FUNCTION_BLOCK FB_SeparatingModule EXTENDS FB_Module
// Module to separate via sensor, barrier and clamp cylinder and axis
VAR_INPUT
		(***** Information about the state and mode of machine *****)
	bExecute					: BOOL;
	bSemiStart					: BOOL;
		(****** Variables to enable / disable diagnosis and temperature mode ******)
	bClampDiag					: BOOL;
	bClampTemp					: BOOL;
	bClampRecord				: BOOL;
	bBarrierDiag				: BOOL;
	bBarrierTemp				: BOOL;
	bBarrierRecord				: BOOL;
		(***** Timer values for clamp and barrier cylinder *****)
	tTimeOutClamp				: TIME;
	tTimeOutBarrier				: TIME;
	tRecordIntervallClamp		: TIME;
	tRecordIntervallBarrier		: TIME;
	tBarrierAtWork				: TIME;
		(***** Information about number of boxes being sorted *****)
	iBoxesOnTheWay				: INT;
		(***** Buttons *****)
	bButtonClampToWorkIn		: BOOL;
	bButtonClampToBaseIn		: BOOL;
	bButtonBarrierToWorkIn		: BOOL;
	bButtonBarrierToBaseIn		: BOOL;
END_VAR
VAR_OUTPUT
	bClampToWork				: BOOL;
	bClampAtBase				: BOOL;
	bClampAtWork				: BOOL;
	bBarrierToWork				: BOOL;
	bBarrierAtBase				: BOOL;
	bBarrierAtWork				: BOOL;
	bClampError					: BOOL;
	sClampErrorMsg				: STRING;
	bBarrierError				: BOOL;
	sBarrierErrorMsg			: STRING;
	aClampTemps					: ARRAY[1..100] OF LREAL;
	aBarrierTemps				: ARRAY[1..100] OF LREAL;
	bSeparated					: BOOL;
	bButtonClampToWorkOut		: BOOL;
	bButtonClampToBaseOut		: BOOL;
	bButtonBarrierToWorkOut		: BOOL;
	bButtonBarrierToBaseOut		: BOOL;
END_VAR
VAR
(* ================= Function block and interface instances ===================== *)
	
	fbSensor					: FB_SignalHandling;
	
		(* Instances of clamp cylinder function blocks *)
	fbClamp						: FB_Cylinder;					// Without diagnosis and temperature mode
	fbClampDiag					: FB_CylinderDiag;				// With diagnosis of states
	fbClampTemp					: FB_CylinderTemp;				// With temperature mode
	fbClampTempDiag				: FB_CylinderTempDiag;			// With diagnosis of temperature
	fbClampTempRecord			: FB_CylinderTempRecord;		// With record of temperatures
		(* Interface instance of ICylinder for clamp cylinder *)
	iClamp						: ICylinder;
	
			(* Instances of barrier cylinder function blocks *)
	fbBarrier					: FB_Cylinder;					// Without diagnosis and temperature mode
	fbBarrierDiag				: FB_CylinderDiag;				// With diagnosis of states
	fbBarrierTemp				: FB_CylinderTemp;				// With temperature mode
	fbBarrierTempDiag			: FB_CylinderTempDiag;			// With diagnosis of temperature
	fbBarrierTempRecord			: FB_CylinderTempRecord;		// With record of temperatures
		(* Interface instance of ICylinder for barrier cylinder *)
	iBarrier					: ICylinder;
	
				(***** Manual cylinder control *****)
	fbButtonClampToWork			: FB_SignalHandlingIntern;		// To move manually clamp cylinder to work position
	fbButtonClampToBase			: FB_SignalHandlingIntern;		// To move manually clamp cylinder to base position
	fbButtonBarrierToWork		: FB_SignalHandlingIntern;		// To move manually barrier cylinder to work position
	fbButtonBarrierToBase		: FB_SignalHandlingIntern;		// To move manually barrier cylinder to base position
	
(* ========================== COMMON VARIABLES =============================== *)	
	fbTimerBarrierAtWork		: TON;							// Timer for opening barrier in AUTOMATIC mode
	eStateAuto					: E_StateSeparatingAuto;
	eStateSemiAuto				: E_StateSeparatingAuto;
END_VAR

// =========================================================
;
// =========================================================

METHOD PROTECTED M_ResetState
VAR_INPUT
END_VAR
// =========================================================

eStateAuto 		:= eSeparatingAuto_Init;
eStateSemiAuto	:= eSeparatingAuto_Init;

// =========================================================
END_METHOD

METHOD PUBLIC M_Semiautomatic
VAR_INPUT
END_VAR
// =========================================================
	// Noticing work position of barrier cylinder	

fbTimerBarrierAtWork( PT := tBarrierAtWork );

// =========================================================
	// Control of main axis

IF iBoxesOnTheWay = 0 AND eStateSemiAuto = eSeparatingAuto_Init THEN
	bHalt := TRUE;
	M_Stop();
END_IF

IF bHalt THEN
	IF bHaltDone THEN
		bHalt := FALSE;
	END_IF
	
	M_Stop();
ELSE
	fbAxis.M_MoveFw();
END_IF

// =========================================================
	// Process of separating boxes
	
CASE eStateSemiAuto OF
	// =========================================================
	eSeparatingAuto_Init:
	
			iBarrier.M_MoveToBase();					(***** Calling method of FB via interface *****)
			
			IF iBarrier.P_AtBasePos						(***** Accessing property of FB via interface *****)
			AND bExecute AND bSemiStart THEN
				eStateSemiAuto := eSeparatingAuto_Start;
			END_IF
		
	// =========================================================
	eSeparatingAuto_Start:
	
			IF fbSensor.bOut THEN
				eStateSemiAuto := eSeparatingAuto_CloseClamp;
			ELSE
				IF NOT iClamp.P_AtWorkPos THEN			(***** Accessing property of FB via interface instance *****)
					iClamp.M_MoveToWork();				(***** Calling method of FB via interface instance *****)
				END_IF
				
				fbAxis.M_MoveFw();
			END_IF
		
	// =========================================================
	eSeparatingAuto_CloseClamp:
	
			iClamp.M_MoveToBase();						(***** Calling method of FB via interface instance *****)
			
			IF iClamp.P_AtBasePos THEN					(***** Accessing property of FB via interface instance *****)
				bSeparated 		:= TRUE;
				eStateSemiAuto 	:= eSeparatingAuto_OpenBarrier;
			END_IF
		
	// =========================================================
	eSeparatingAuto_OpenBarrier:
	
			iBarrier.M_MoveToWork();					(***** Calling method of FB via interface *****)
			
			IF iBarrier.P_AtWorkPos THEN				(***** Accessing property of FB via interface *****)
				fbTimerBarrierAtWork( IN := TRUE );
			END_IF
			
			IF fbTimerBarrierAtWork.Q THEN
				fbTimerBarrierAtWork( IN := FALSE );
				eStateSemiAuto := eSeparatingAuto_CloseBarrier;
			END_IF
		
	// =========================================================
	eSeparatingAuto_CloseBarrier:
	
			iBarrier.M_MoveToBase();					(***** Calling method of FB via interface *****)
			
			IF iBarrier.P_AtBasePos THEN				(***** Accessing property of FB via interface *****)
				bSeparated 		:= FALSE;
				eStateSemiAuto 	:= eSeparatingAuto_OpenClamp;
			END_IF
		
	// =========================================================
	eSeparatingAuto_OpenClamp:
	
			iClamp.M_MoveToWork();						(***** Calling method of FB via interface instance *****)
			
			IF iClamp.P_AtWorkPos THEN					(***** Accessing property of FB via interface instance *****)
				eStateSemiAuto := eSeparatingAuto_Init;
			END_IF
END_CASE

// =========================================================
END_METHOD

METHOD PUBLIC M_SetOutput
VAR_INPUT
END_VAR
// =========================================================
		// Calling method M_SetOutput of base class FB_Module via 'SUPER^.'
		
SUPER^.M_SetOutput();						

// =========================================================
		// Sensor
		
fbSensor.M_SetOutput();

// =========================================================
		// Cylinder buttons
		
fbButtonClampToWork.M_SetOutput();
fbButtonClampToBase.M_SetOutput();
fbButtonBarrierToWork.M_SetOutput();
fbButtonBarrierToBase.M_SetOutput();

// =========================================================
		// Output variables for cylinders
		
bClampToWork 	:= iClamp.P_ToWork;			// Assigning global output variable to property of selected FB
											// Accessing property of selected FB via interface instance
bClampAtWork 	:= iClamp.P_AtWorkPos;
bClampAtBase 	:= iClamp.P_AtBasePos;
		
bBarrierToWork 	:= iBarrier.P_ToWork;		// Assigning global output variable to property of selected FB
											// Accessing property of selected FB via interface instance
bBarrierAtWork 	:= iBarrier.P_AtWorkPos;
bBarrierAtBase	:= iBarrier.P_AtBasePos;

// =========================================================
		// Buttons

fbButtonClampToWork.bInput 		:= bButtonClampToWorkIn;
fbButtonClampToBase.bInput 		:= bButtonClampToBaseIn;
fbButtonBarrierToWork.bInput 	:= bButtonBarrierToWorkIn;
fbButtonBarrierToBase.bInput 	:= bButtonBarrierToBaseIn;
bButtonClampToWorkOut 			:= fbButtonClampToWork.bOut;
bButtonClampToBaseOut 			:= fbButtonClampToBase.bOut;
bButtonBarrierToWorkOut 		:= fbButtonBarrierToWork.bOut;
bButtonBarrierToBaseOut 		:= fbButtonBarrierToBase.bOut;

// =========================================================
END_METHOD

METHOD PUBLIC M_Manual
VAR_INPUT
END_VAR
// =========================================================
	// Calling method M_Manual of base class FB_Module via 'SUPER^.'
		
SUPER^.M_Manual();							

// =========================================================
	// Manual cylinder control
	
IF fbButtonClampToWork.bOut THEN
	iClamp.M_MoveToWork();					(**** Calling method of FB via interface instance ****)
	
ELSIF fbButtonClampToBase.bOut THEN
	iClamp.M_MoveToBase();					(**** Calling method of FB via interface instance ****)
END_IF

IF fbButtonBarrierToWork.bOut THEN
	iBarrier.M_MoveToWork();				(**** Calling method of FB via interface instance ****)
	
ELSIF fbButtonBarrierToBase.bOut THEN
	iBarrier.M_MoveToBase();				(**** Calling method of FB via interface instance ****)
END_IF

// =========================================================
END_METHOD

METHOD PUBLIC M_Reset
VAR_INPUT
END_VAR
// =========================================================
		// Resetting cylinder and axis
		
fbTriggerResetStart( CLK := bReset );

IF fbTriggerResetStart.Q THEN
	bSeparated := FALSE;
	
	fbTimerBarrierAtWork( IN := FALSE );
	iClamp.M_Reset();					(**** Calling method of FB via interface ****)
	iBarrier.M_Reset();					(**** Calling method of FB via interface ****)
END_IF

// =========================================================
		// Calling method of base class
		
SUPER^.M_Reset();						// Calling method M_Reset of base class FB_Module via 'SUPER^.'

// =========================================================
END_METHOD

METHOD PUBLIC M_Maintenance
VAR_INPUT
END_VAR
// =========================================================
	// Calling own method M_Manual of this class FB_SeparatingModule via 'THIS^.'
		
THIS^.M_Manual();				

// =========================================================
END_METHOD

METHOD PUBLIC M_Enable
VAR_INPUT
END_VAR
// =========================================================
		// Calling method M_Enable of base class FB_Module via 'SUPER^.'
		
SUPER^.M_Enable();

// =========================================================
		// Sensor control
		
fbSensor.bEnable := bSensorEnable;

// =========================================================
		// Cylinder control
		
fbButtonClampToWork.bEnable		:= bManualCylinderEnable
									AND NOT iClamp.P_AtWorkPos;		(*** Accessing property of FB via interface instance ***)
								
fbButtonClampToBase.bInput 		:= NOT fbButtonClampToWork.bInput;

fbButtonClampToBase.bEnable 	:= bManualCylinderEnable
									AND NOT iClamp.P_AtBasePos;		(*** Accessing property of FB via interface instance ***)

fbButtonBarrierToWork.bEnable 	:= bManualCylinderEnable
									AND NOT iBarrier.P_AtWorkPos;	(*** Accessing property of FB via interface instance ***)
								
fbButtonBarrierToBase.bInput 	:= NOT fbButtonBarrierToWork.bInput;

fbButtonBarrierToBase.bEnable 	:= bManualCylinderEnable
									AND NOT iBarrier.P_AtBasePos;	(*** Accessing property of FB via interface instance ***)

// =========================================================
END_METHOD

METHOD PUBLIC M_CylinderOptions
VAR_INPUT
END_VAR
// =========================================================
		// Selecting clamp cylinder

// Checking variables to enable / disable diagnosis and temperature mode
IF bClampDiag THEN
	IF bClampTemp THEN
		
	(* ============== FB with diagnosis and temperature mode ============== *)
		bClampError 	:= fbClampTempDiag.bError;			// Assigning global output variable to output variable of selected FB
		sClampErrorMsg 	:= fbClampTempDiag.sErrorMsg;
		iClamp 			:= fbClampTempDiag;					// Assigning desired FB instance to interface instance
	
	ELSE
	
	(* ============== FB with diagnosis and without temperature mode ============== *)
		fbClampDiag.tTimeOut 	:= tTimeOutClamp;			// Setting special data for selected FB
		bClampError 			:= fbClampDiag.bError;		// Assigning global output variable to output variable of selected FB
		sClampErrorMsg 			:= fbClampDiag.sErrorMsg;
		iClamp 					:= fbClampDiag;				// Assigning desired FB instance to interface instance
	END_IF
ELSE
	bClampError := FALSE;
	sClampErrorMsg := '';
	
	IF bClampTemp THEN
		IF bClampRecord THEN
			fbClampTempRecord.tIntervalTime 	:= tRecordIntervallClamp;	// Time of record interval
			fbClampTempRecord.bRecordStart 		:= bComprAirEnabled;		// Recording if compressed air is set
			
			fbClampTempRecord.M_Record();									// Calling method of function block FB_CylinderTempRecord
			
			aClampTemps 	:= fbClampTempRecord.aTemps;					// Saving output variable
			iClamp 			:= fbClampTempRecord;
		ELSE
			(* ============== FB without diagnosis and with temperature mode ============== *)
			iClamp := fbClampTemp; 						// Assigning desired FB instance to interface instance
		END_IF
	ELSE
	
	(* ============== FB without diagnosis and temperature mode ============== *)
		iClamp := fbClamp;							// Assigning desired FB instance to interface instance						
	END_IF	
END_IF
									
// =========================================================
// =========================================================
			(**** Selecting barrier cylinder ****)

// Checking variables to enable / disable diagnosis and temperature mode
IF bBarrierDiag THEN
	IF bBarrierTemp THEN
		
	(* ============== FB with diagnosis and temperature mode ============== *)
		bBarrierError 		:= fbBarrierTempDiag.bError;		// Assigning global output variable to output variable of selected FB
		sBarrierErrorMsg 	:= fbBarrierTempDiag.sErrorMsg;
		iBarrier 			:= fbBarrierTempDiag;				// Assigning desired FB instance to interface instance
	
	ELSE
	
	(* ============== FB with diagnosis and without temperature mode ============== *)
		fbBarrierDiag.tTimeOut	:= tTimeOutBarrier;				// Setting special data for selected FB
		bBarrierError 			:= fbBarrierDiag.bError;		// Assigning global output variable to output variable of selected FB
		sBarrierErrorMsg 		:= fbBarrierDiag.sErrorMsg;
		iBarrier 				:= fbBarrierDiag;				// Assigning desired FB instance to interface instance
	END_IF
ELSE
	bBarrierError := FALSE;
	sBarrierErrorMsg := '';
	
	IF bBarrierTemp THEN
		IF bBarrierRecord THEN
			fbBarrierTempRecord.tIntervalTime 	:= tRecordIntervallBarrier;		// Time of record interval
			fbBarrierTempRecord.bRecordStart 	:= bComprAirEnabled;			// Recording if compressed air is set
			
			fbBarrierTempRecord.M_Record();										// Calling method of function block FB_CylinderTempRecord
			
			aBarrierTemps 	:= fbBarrierTempRecord.aTemps;						// Saving output variable
			iBarrier 		:= fbBarrierTempRecord;
		ELSE
			(* ============== FB without diagnosis and with temperature mode ============== *)
			iBarrier := fbBarrierTemp; 						// Assigning desired FB instance to interface instance
		END_IF
	ELSE
	
	(* ============== FB without diagnosis and temperature mode ============== *)
		iBarrier := fbBarrier;							// Assigning desired FB instance to interface instance						
	END_IF	
END_IF
									
// =========================================================
END_METHOD

METHOD PUBLIC M_Automatic
VAR_INPUT
END_VAR
// =========================================================
	// Noticing work position of barrier cylinder	

fbTimerBarrierAtWork( PT := tBarrierAtWork );

// =========================================================
	// Control of main axis

IF NOT bHalt THEN
	fbAxis.M_MoveFw();
	
ELSIF NOT bHaltDone THEN
	M_Stop();
	
ELSE
	bHalt := FALSE;
	M_Stop();
END_IF

// =========================================================
	// Process of separating boxes
	
CASE eStateAuto OF
	// =========================================================
	eSeparatingAuto_Init:
	
			iBarrier.M_MoveToBase();					(***** Calling method of FB via interface *****)
			
			IF iBarrier.P_AtBasePos AND bExecute THEN	(***** Accessing property of FB via interface *****)
				eStateAuto := eSeparatingAuto_Start;
			END_IF
		
	// =========================================================
	eSeparatingAuto_Start:
	
			IF fbSensor.bOut AND fbAxis.bMoves THEN
				eStateAuto := eSeparatingAuto_CloseClamp;
				
			ELSIF NOT iClamp.P_AtWorkPos THEN			(***** Accessing property of FB via interface instance *****)
				iClamp.M_MoveToWork();					(***** Calling method of FB via interface instance *****)
			END_IF
		
	// =========================================================
	eSeparatingAuto_CloseClamp:
	
			iClamp.M_MoveToBase();						(***** Calling method of FB via interface instance *****)
			
			IF iClamp.P_AtBasePos THEN					(***** Accessing property of FB via interface instance *****)
				bSeparated 	:= TRUE;
				eStateAuto 	:= eSeparatingAuto_OpenBarrier;
			END_IF
		
	// =========================================================
	eSeparatingAuto_OpenBarrier:
	
			iBarrier.M_MoveToWork();					(***** Calling method of FB via interface *****)
			
			IF iBarrier.P_AtWorkPos THEN				(***** Accessing property of FB via interface *****)
				fbTimerBarrierAtWork( IN := TRUE );
			END_IF
			
			IF fbTimerBarrierAtWork.Q THEN
				fbTimerBarrierAtWork( IN := FALSE );
				eStateAuto := eSeparatingAuto_CloseBarrier;
			END_IF
		
	// =========================================================
	eSeparatingAuto_CloseBarrier:
	
			iBarrier.M_MoveToBase();					(***** Calling method of FB via interface *****)
			
			IF iBarrier.P_AtBasePos THEN				(***** Accessing property of FB via interface *****)
				bSeparated 	:= FALSE;
				eStateAuto	:= eSeparatingAuto_OpenClamp;
			END_IF
		
	// =========================================================
	eSeparatingAuto_OpenClamp:
	
			iClamp.M_MoveToWork();						(***** Calling method of FB via interface instance *****)
			
			IF iClamp.P_AtWorkPos THEN					(***** Accessing property of FB via interface instance *****)
				eStateAuto := eSeparatingAuto_Init;
			END_IF
END_CASE

// =========================================================
END_METHOD

END_FUNCTION_BLOCK
